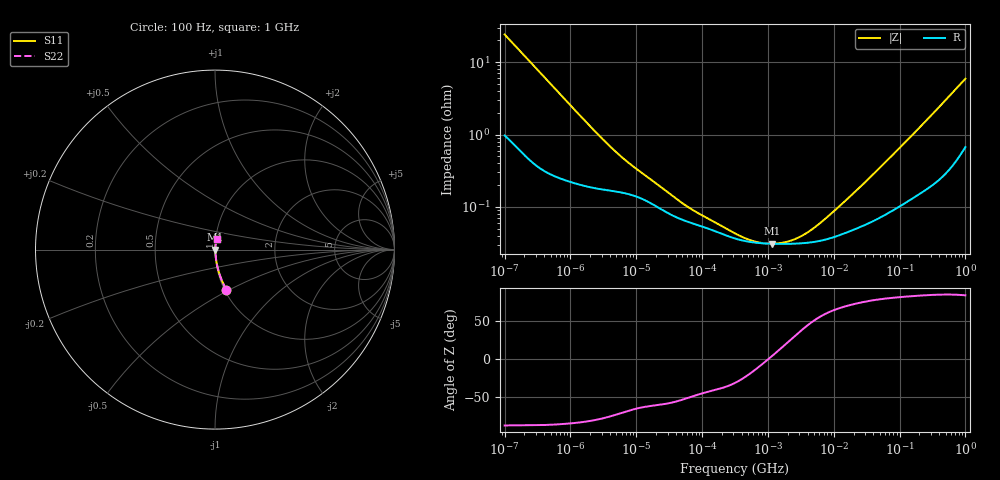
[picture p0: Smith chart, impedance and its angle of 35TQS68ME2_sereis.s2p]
!  *** S-Parameter ***
!  Copyright (C) Panasonic Industry
!  Conductive Polymer Tantalum Solid Capacitor (POSCAP)
!  Parts No. 35TQS68ME2
!  Connection Mode : Series
!  1  o---||---o  2
!  GND o--------o GND
!  Conditions : Temperature = 20   DC Bias = 0 V
! Frequency Range : 100 Hz  -  1 GHz  [ 401 Steps ]
# Hz S RI R 50
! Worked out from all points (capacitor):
!   401 points, 100 Hz to 1 GHz, reference 50 ohm
!   read as one part in series: C = 65.4 uF near 108.4 Hz
!   lowest |Z| = 31 mohm at 1.148 MHz (marker M1)
!   series resonance near 1.031 MHz, so ESL is about 360 pH
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100  0.0631 -0.2238  0.9369 0.2238  0.9369 0.2238  0.0631 -0.2238
183.0206  0.0229 -0.1301  0.9771 0.1301  0.9771 0.1301  0.0229 -0.1301
321.7363  0.00937 -0.0759  0.9906 0.0759  0.9906 0.0759  0.00937 -0.0759
638.2635  0.00406 -0.0389  0.9959 0.0389  0.9959 0.0389  0.00406 -0.0389
1487.647  0.00228 -0.017  0.9977 0.017  0.9977 0.017  0.00228 -0.017
3198.895  0.00179 -0.00816  0.9982 0.00816  0.9982 0.00816  0.00179 -0.00816
5623.413  0.00162 -0.00488  0.9984 0.00488  0.9984 0.00488  0.00162 -0.00488
9120.108  0.00144 -0.00328  0.9986 0.00328  0.9986 0.00328  0.00144 -0.00328
22130.95  0.000969 -0.00171  0.999 0.00171  0.999 0.00171  0.000969 -0.00171
65690.11  0.000608 -0.000736  0.9994 0.000736  0.9994 0.000736  0.000608 -0.000736
316227.8  0.000366 -0.000226  0.9996 0.000226  0.9996 0.000226  0.000366 -0.000226
602559.6  0.000323 -9.36e-05  0.9997 9.36e-05  0.9997 9.36e-05  0.000323 -9.36e-05
1148154  0.000309 1.85e-05  0.9997 -1.85e-05  0.9997 -1.85e-05  0.000309 1.85e-05
1650061  0.000308 8.37e-05  0.9997 -8.37e-05  0.9997 -8.37e-05  0.000308 8.37e-05
2371374  0.000309 0.00016  0.9997 -0.00016  0.9997 -0.00016  0.000309 0.00016
3273407  0.000314 0.000244  0.9997 -0.000244  0.9997 -0.000244  0.000314 0.000244
4704354  0.000325 0.000368  0.9997 -0.000368  0.9997 -0.000368  0.000325 0.000368
7328245  0.000352 0.000579  0.9996 -0.000579  0.9996 -0.000579  0.000352 0.000579
1.513561e7  0.000438 0.00114  0.9996 -0.00114  0.9996 -0.00114  0.000438 0.00114
6.99842e7  0.000858 0.00462  0.9991 -0.00462  0.9991 -0.00462  0.000858 0.00462
3.368992e8  0.00249 0.0202  0.9975 -0.0202  0.9975 -0.0202  0.00249 0.0202
1e9  0.01 0.0578  0.99 -0.0578  0.99 -0.0578  0.01 0.0578
